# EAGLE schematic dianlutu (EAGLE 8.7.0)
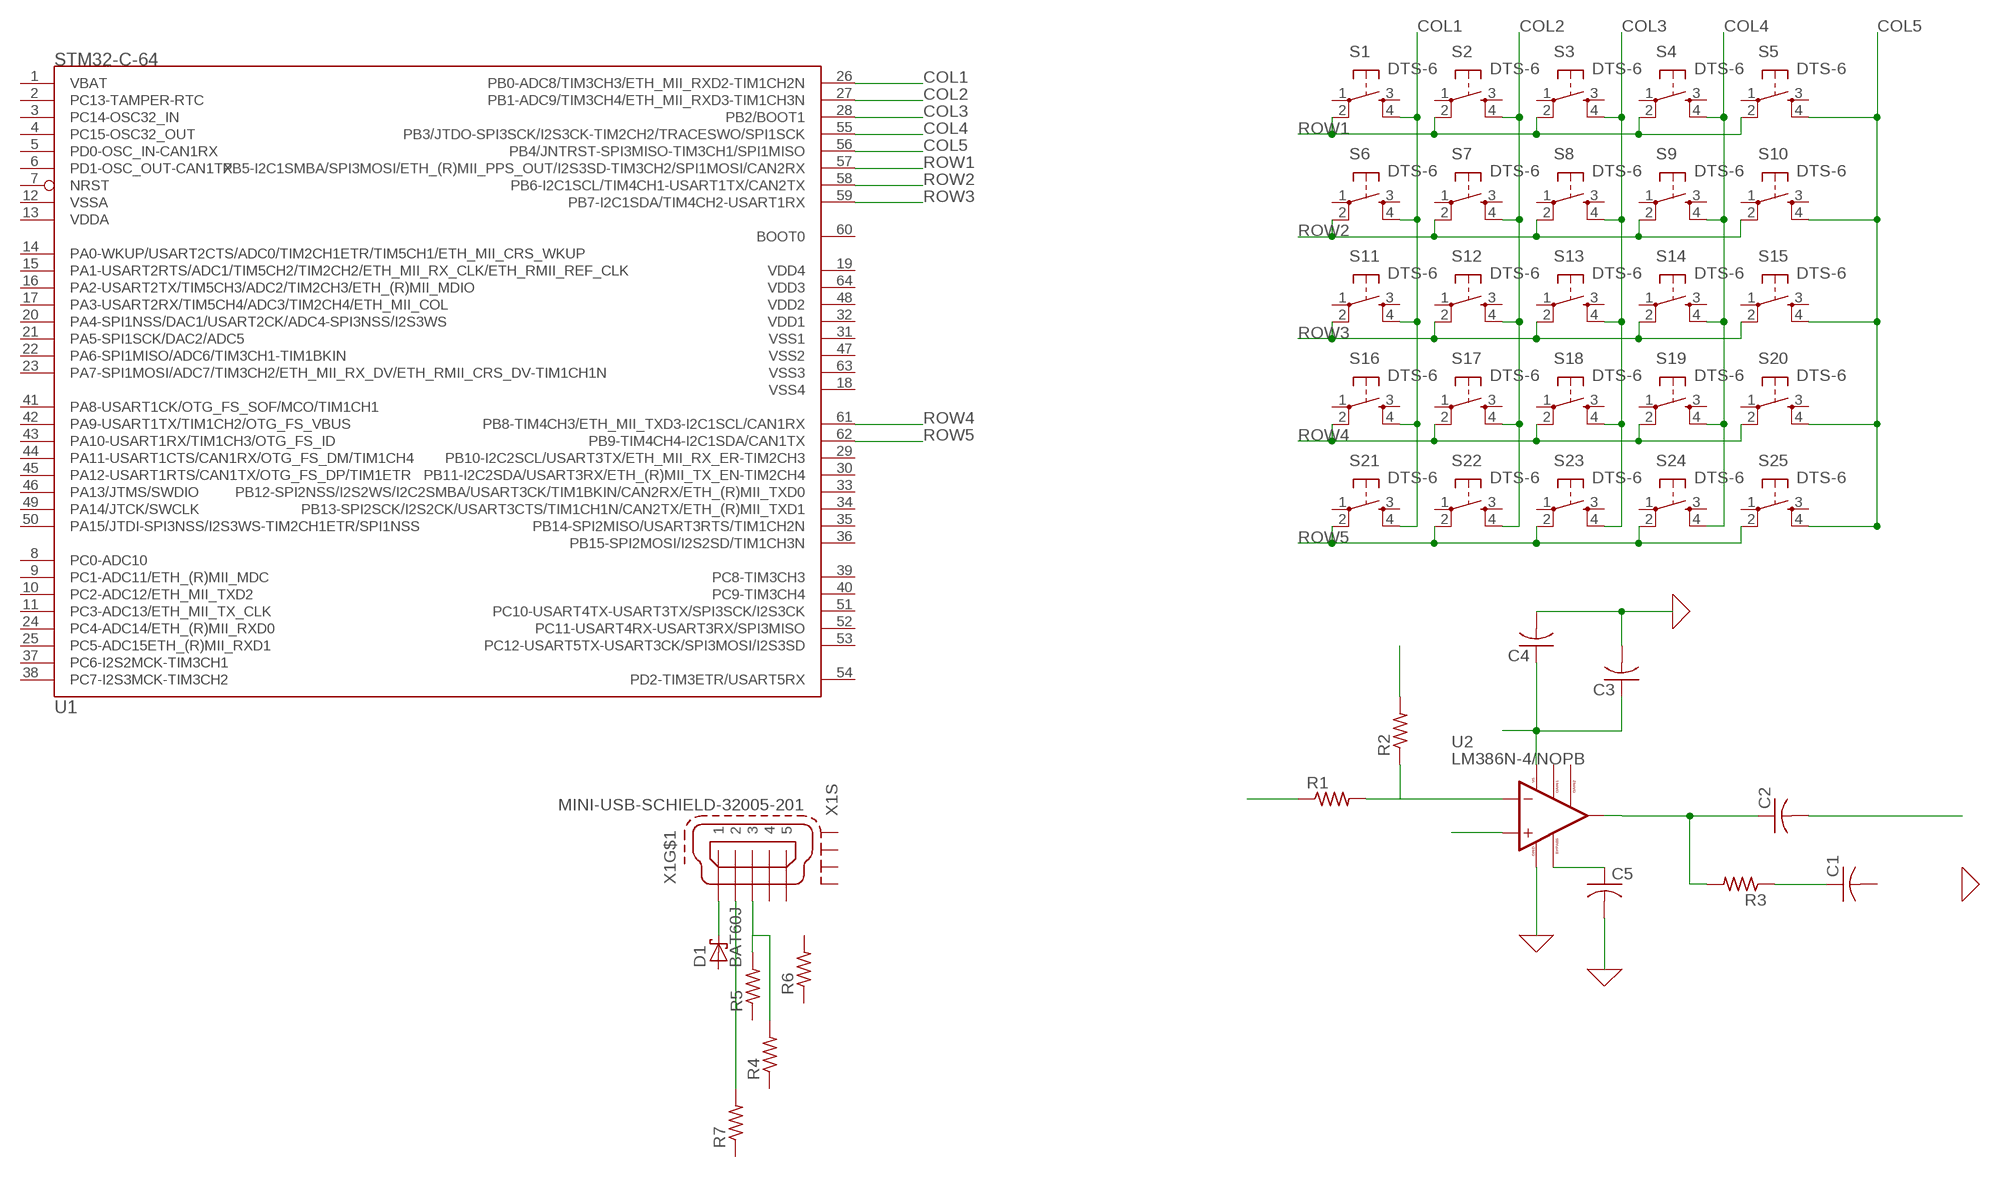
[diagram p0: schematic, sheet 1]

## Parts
C1  C-USC0805  [C0805]
C2  C-USC0805  [C0805]
C3  C-USC0805  [C0805]
C4  C-USC0805  [C0805]
C5  C-USC0805  [C0805]
D1  BAT60J  [SOD323_ST]
R1  R-US_R0805  [R0805]
R2  R-US_R0805  [R0805]
R3  R-US_R0805  [R0805]
R4  R-US_M0805  [M0805]
R5  R-US_M0805  [M0805]
R6  R-US_M0805  [M0805]
R7  R-US_M0805  [M0805]
S1  DTS-6  [DTS-6]
S2  DTS-6  [DTS-6]
S3  DTS-6  [DTS-6]
S4  DTS-6  [DTS-6]
S5  DTS-6  [DTS-6]
S6  DTS-6  [DTS-6]
S7  DTS-6  [DTS-6]
S8  DTS-6  [DTS-6]
S9  DTS-6  [DTS-6]
S10  DTS-6  [DTS-6]
S11  DTS-6  [DTS-6]
S12  DTS-6  [DTS-6]
S13  DTS-6  [DTS-6]
S14  DTS-6  [DTS-6]
S15  DTS-6  [DTS-6]
S16  DTS-6  [DTS-6]
S17  DTS-6  [DTS-6]
S18  DTS-6  [DTS-6]
S19  DTS-6  [DTS-6]
S20  DTS-6  [DTS-6]
S21  DTS-6  [DTS-6]
S22  DTS-6  [DTS-6]
S23  DTS-6  [DTS-6]
S24  DTS-6  [DTS-6]
S25  DTS-6  [DTS-6]
U1  STM32-C-64  [LQFP64]
U2  LM386N-4/NOPB  [DIP794W45P254L1016H508Q8]
X1  MINI-USB-SCHIELD-32005-201  [32005-201]

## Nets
0: C3.2 C4.2 C5.2 U2.4(GND) ; supply symbol labelled GND
COL1: S1.4 S6.4 S11.4 S16.4 S21.4 U1.26(PB0-ADC8/TIM3CH3/ETH_MII_RXD2-TIM1CH2N)
COL2: S2.4 S7.4 S12.4 S17.4 S22.4 U1.27(PB1-ADC9/TIM3CH4/ETH_MII_RXD3-TIM1CH3N)
COL3: S3.4 S8.4 S13.4 S18.4 S23.4 U1.28(PB2/BOOT1)
COL4: S4.4 S9.4 S14.4 S19.4 S24.4 U1.55(PB3/JTDO-SPI3SCK/I2S3CK-TIM2CH2/TRACESWO/SPI1SCK)
COL5: S5.4 S10.4 S15.4 S20.4 S25.4 U1.56(PB4/JNTRST-SPI3MISO-TIM3CH1/SPI1MISO)
N$1: D1.C X1.1
N$2: R7.2 X1.2
N$3: R4.2 R5.2 X1.3
N$11: R1.2 R2.1 U2.2(-INPUT)
N$12: U2.3(+INPUT)
N$13: R1.1
N$14: R2.2
N$16: C5.1
N$18: C2.1 R3.2 U2.5(VOUT)
N$20: C3.1 C4.1 U2.6(VS)
N$22: C1.1 R3.1
N$23: C2.2
ROW1: S1.2 S2.2 S3.2 S4.2 S5.2 U1.57(PB5-I2C1SMBA/SPI3MOSI/ETH_(R)MII_PPS_OUT/I2S3SD-TIM3CH2/SPI1MOSI/CAN2RX)
ROW2: S6.2 S7.2 S8.2 S9.2 S10.2 U1.58(PB6-I2C1SCL/TIM4CH1-USART1TX/CAN2TX)
ROW3: S11.2 S12.2 S13.2 S14.2 S15.2 U1.59(PB7-I2C1SDA/TIM4CH2-USART1RX)
ROW4: S16.2 S17.2 S18.2 S19.2 S20.2 U1.61(PB8-TIM4CH3/ETH_MII_TXD3-I2C1SCL/CAN1RX)
ROW5: S21.2 S22.2 S23.2 S24.2 S25.2 U1.62(PB9-TIM4CH4-I2C1SDA/CAN1TX)
Unconnected: C1.2 D1.A R4.1 R5.1 R6.1 R6.2 R7.1 S1.1 S1.3 S2.1 S2.3 S3.1 S3.3 S4.1 S4.3 S5.1 S5.3 S6.1 S6.3 S7.1 S7.3 S8.1 S8.3 S9.1 S9.3 S10.1 S10.3 S11.1 S11.3 S12.1 S12.3 S13.1 S13.3 S14.1 S14.3 S15.1 S15.3 S16.1 S16.3 S17.1 S17.3 S18.1 S18.3 S19.1 S19.3 S20.1 S20.3 S21.1 S21.3 S22.1 S22.3 S23.1 S23.3 S24.1 S24.3 S25.1 S25.3 U1.1(VBAT) U1.2(PC13-TAMPER-RTC) U1.3(PC14-OSC32_IN) U1.4(PC15-OSC32_OUT) U1.5(PD0-OSC_IN-CAN1RX) U1.6(PD1-OSC_OUT-CAN1TX) U1.7(NRST) U1.8(PC0-ADC10) U1.9(PC1-ADC11/ETH_(R)MII_MDC) U1.10(PC2-ADC12/ETH_MII_TXD2) U1.11(PC3-ADC13/ETH_MII_TX_CLK) U1.12(VSSA) U1.13(VDDA) U1.14(PA0-WKUP/USART2CTS/ADC0/TIM2CH1ETR/TIM5CH1/ETH_MII_CRS_WKUP) U1.15(PA1-USART2RTS/ADC1/TIM5CH2/TIM2CH2/ETH_MII_RX_CLK/ETH_RMII_REF_CLK) U1.16(PA2-USART2TX/TIM5CH3/ADC2/TIM2CH3/ETH_(R)MII_MDIO) U1.17(PA3-USART2RX/TIM5CH4/ADC3/TIM2CH4/ETH_MII_COL) U1.18(VSS4) U1.19(VDD4) U1.20(PA4-SPI1NSS/DAC1/USART2CK/ADC4-SPI3NSS/I2S3WS) U1.21(PA5-SPI1SCK/DAC2/ADC5) U1.22(PA6-SPI1MISO/ADC6/TIM3CH1-TIM1BKIN) U1.23(PA7-SPI1MOSI/ADC7/TIM3CH2/ETH_MII_RX_DV/ETH_RMII_CRS_DV-TIM1CH1N) U1.24(PC4-ADC14/ETH_(R)MII_RXD0) U1.25(PC5-ADC15ETH_(R)MII_RXD1) U1.29(PB10-I2C2SCL/USART3TX/ETH_MII_RX_ER-TIM2CH3) U1.30(PB11-I2C2SDA/USART3RX/ETH_(R)MII_TX_EN-TIM2CH4) U1.31(VSS1) U1.32(VDD1) U1.33(PB12-SPI2NSS/I2S2WS/I2C2SMBA/USART3CK/TIM1BKIN/CAN2RX/ETH_(R)MII_TXD0) U1.34(PB13-SPI2SCK/I2S2CK/USART3CTS/TIM1CH1N/CAN2TX/ETH_(R)MII_TXD1) U1.35(PB14-SPI2MISO/USART3RTS/TIM1CH2N) U1.36(PB15-SPI2MOSI/I2S2SD/TIM1CH3N) U1.37(PC6-I2S2MCK-TIM3CH1) U1.38(PC7-I2S3MCK-TIM3CH2) U1.39(PC8-TIM3CH3) U1.40(PC9-TIM3CH4) U1.41(PA8-USART1CK/OTG_FS_SOF/MCO/TIM1CH1) U1.42(PA9-USART1TX/TIM1CH2/OTG_FS_VBUS) U1.43(PA10-USART1RX/TIM1CH3/OTG_FS_ID) U1.44(PA11-USART1CTS/CAN1RX/OTG_FS_DM/TIM1CH4) U1.45(PA12-USART1RTS/CAN1TX/OTG_FS_DP/TIM1ETR) U1.46(PA13/JTMS/SWDIO) U1.47(VSS2) U1.48(VDD2) U1.49(PA14/JTCK/SWCLK) U1.50(PA15/JTDI-SPI3NSS/I2S3WS-TIM2CH1ETR/SPI1NSS) U1.51(PC10-USART4TX-USART3TX/SPI3SCK/I2S3CK) U1.52(PC11-USART4RX-USART3RX/SPI3MISO) U1.53(PC12-USART5TX-USART3CK/SPI3MOSI/I2S3SD) U1.54(PD2-TIM3ETR/USART5RX) U1.60(BOOT0) U1.63(VSS3) U1.64(VDD3) U2.1(GAIN1) U2.7(BYPASS) U2.8(GAIN2) X1.4 X1.5 X1.M1(S:S1) X1.M2(S:S2) X1.M3(S:S3) X1.M4(S:S4)

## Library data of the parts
C1-C5 = rcl:C-US: CAPACITOR, American symbol; SPICEPREFIX: C
D1 = diode:BAT60J: Schottky barrier diode
R1-R3 = rcl:R-US_: RESISTOR, American symbol; SPICEPREFIX: R
R4-R7 = resistor:R-US_: RESISTOR, American symbol
S1-S25 = switch-tact:DTS-6
U1 = pel_stm32:STM32-C-64
U2 = LM386N-4_NOPB:LM386N-4/NOPB: Linear IC - Audio amplifier Texas Instruments LM386N-4/NOPB 1-channel (mono) Class AB PDIP 8; AVAILABILITY: Unavailable; DESCRIPTION: Linear IC - Audio amplifier Texas Instruments LM386N-4/NOPB 1-channel _mono_ Class AB PDIP 8; MF: Texas Instruments; MP: LM386N-4/NOPB; PACKAGE: DIP-8 Texas Instruments; PRICE: None
X1 = con-cypressindustries:MINI-USB-SCHIELD-: MINI USB-B Conector Source: www.cypressindustries.com; OC_FARNELL: unknown; OC_NEWARK: unknown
